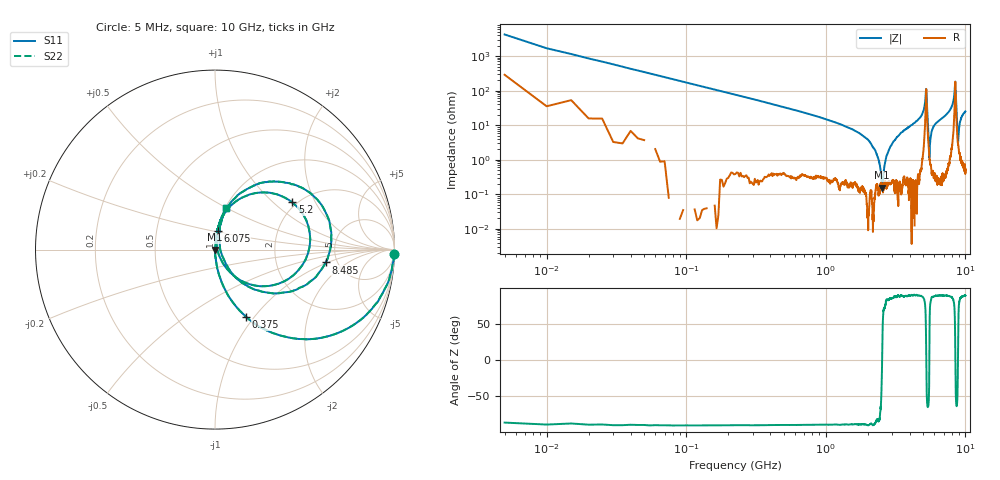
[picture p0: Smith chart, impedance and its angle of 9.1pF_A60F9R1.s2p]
! Amotech Co.,Ltd.
! http://www.amotech.co.kr/
! Part Number: A60F9R1
! These Parameters are Measured in Series Mode Connection
! Operation Temp=25[degC], DC Bias Voltage=0[V]
! Freq. Start=5[MHz] Stop=10[GHz], 2000[Steps]
! Date: Monday, July 20, 2020, 04:05:45
# GHZ S RI R 50.000000
!Freq.(Hz) S11(Real) S11(Imag) S21(Real) S21(Imag) S12(Real) S12(Imag) S22(Real) S22(Imag)
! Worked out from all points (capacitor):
!   2000 points, 5 MHz to 10 GHz, reference 50 ohm
!   read as one part in series: C = 9.2 pF near 55 MHz
!   lowest |Z| = 156 mohm at 2.535 GHz (marker M1)
!   series resonance near 2.531 GHz, so ESL is about 430 pH
!   S11 on the Smith chart (normalised r, x): 5 MHz: 7, -85; 375 MHz: 1.01, -0.91; 5.2 GHz: 1.90, +1.34; 6.075 GHz: 1.01, +0.21; 8.485 GHz: 4.05, -0.94; 10 GHz: 1.01, +0.50
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0.005  0.9978 -0.0235  0.00215 0.0235  0.00215 0.0235  0.9978 -0.0235
0.11  0.7113 -0.4533  0.2887 0.4533  0.2887 0.4533  0.7113 -0.4533
0.375  0.172 -0.374  0.828 0.374  0.828 0.374  0.172 -0.374
1.675  0.00579 -0.0631  0.9942 0.0631  0.9942 0.0631  0.00579 -0.0631
2.27  0.00164 -0.0178  0.9984 0.0178  0.9984 0.0178  0.00164 -0.0178
2.535  0.00155 0.000194  0.9985 -0.000194  0.9985 -0.000194  0.00155 0.000194
2.77  0.00218 0.015  0.9978 -0.015  0.9978 -0.015  0.00218 0.015
3.34  0.00467 0.0509  0.9953 -0.0509  0.9953 -0.0509  0.00467 0.0509
5.005  0.0776 0.2338  0.9224 -0.2338  0.9224 -0.2338  0.0776 0.2338
5.2  0.4309 0.263  0.5691 -0.263  0.5691 -0.263  0.4309 0.263
5.305  0.231 -0.2016  0.769 0.2016  0.769 0.2016  0.231 -0.2016
5.525  0.0106 0.00557  0.9894 -0.00557  0.9894 -0.00557  0.0106 0.00557
5.725  0.00854 0.0636  0.9915 -0.0636  0.9915 -0.0636  0.00854 0.0636
6.075  0.0145 0.1053  0.9855 -0.1053  0.9855 -0.1053  0.0145 0.1053
6.67  0.025 0.146  0.975 -0.146  0.975 -0.146  0.025 0.146
7.92  0.1057 0.2811  0.8943 -0.2811  0.8943 -0.2811  0.1057 0.2811
8.335  0.4162 0.3695  0.5838 -0.3695  0.5838 -0.3695  0.4162 0.3695
8.485  0.617 -0.0713  0.383 0.0713  0.383 0.0713  0.617 -0.0713
8.65  0.1363 -0.1728  0.8637 0.1728  0.8637 0.1728  0.1363 -0.1728
8.85  0.0282 0.00445  0.9718 -0.00445  0.9718 -0.00445  0.0282 0.00445
9.175  0.0264 0.1241  0.9736 -0.1241  0.9736 -0.1241  0.0264 0.1241
10  0.0628 0.2325  0.9372 -0.2325  0.9372 -0.2325  0.0628 0.2325
